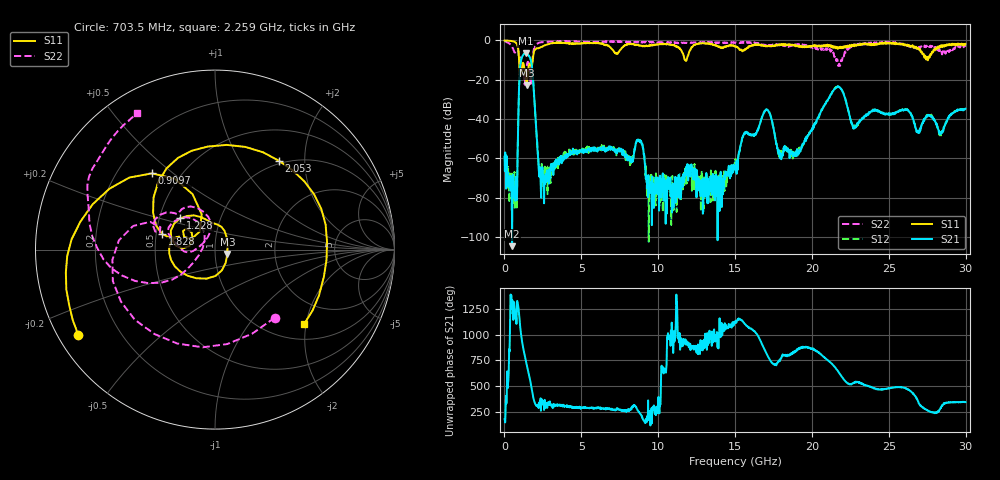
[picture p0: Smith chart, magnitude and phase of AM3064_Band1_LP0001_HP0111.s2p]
# Hz S DB R 50.0
!freq dBS11 angS11 dBS21 angS21 dBS12 angS12 dBS22 angS22
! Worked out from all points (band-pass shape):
!   1600 points, 10 MHz to 29.98 GHz, reference 50 ohm
!   highest |S21| = -6.51 dB at 1.378 GHz (marker M1); lowest = -104.6 dB at 497.3 MHz (marker M2)
!   |S21| within 3 dB of the highest: 1.094 GHz to 1.698 GHz (603.7 MHz wide, 43.2 % of centre)
!   lowest |S11| = -22.7 dB at 1.453 GHz (marker M3), VSWR 1.16, Z = 57.3 - j2.79 ohm
!   |S11| at or under -10 dB: 949.3 MHz to 1.833 GHz (883.2 MHz wide, 63.5 % of centre); 11.74 GHz to 11.84 GHz (102.1 MHz wide, 0.866 % of centre); 27.53434 GHz to 27.54646 GHz (12.12 MHz wide, 0.044 % of centre)
!   |S22| runs from -23.1 to -0.2 dB; largest |S21 - S12| = 0.0045
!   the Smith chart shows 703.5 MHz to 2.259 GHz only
!   S11 on the Smith chart (normalised r, x): 703.5 MHz: 0.06, -0.29; 909.7 MHz: 0.35, +0.42; 1.228 GHz: 0.64, +0.24; 1.828 GHz: 0.54, +0.10; 2.053 GHz: 0.95, +1.50; 2.259 GHz: 1.36, -1.95
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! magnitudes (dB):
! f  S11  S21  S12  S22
! 10 MHz  -0.1  -59.1  -58.7  -0.2
! 497.3 MHz  -0.4  -104.6  -67.3  -3.2
! 703.5 MHz  -0.9  -81.6  -73.1  -5.9
! 909.7 MHz  -5.2  -36.3  -36.2  -6.5
! 1.228 GHz  -11.7  -7.3  -7.3  -13.1
! 1.378 GHz  -17.6  -6.5  -6.5  -16.4
! 1.453 GHz  -22.7  -6.7  -6.7  -12.8
! 1.828 GHz  -10.3  -16.4  -16.3  -9.1
! 2.053 GHz  -4.3  -43.4  -43.3  -2.0
! 2.259 GHz  -3.8  -69.2  -67.0  -1.1
! 5.015 GHz  -1.4  -56.5  -56.1  -0.6
! 8.763 GHz  -2.7  -50.9  -51.0  -1.1
! 10 GHz  -2.0  -78.3  -71.9  -0.9
! 15 GHz  -3.0  -65.8  -63.8  -1.2
! 17.01 GHz  -3.1  -35.2  -35.2  -2.4
! 17.97 GHz  -2.4  -57.8  -58.3  -2.0
! 19.99 GHz  -3.2  -45.9  -45.7  -3.3
! 21.66 GHz  -3.7  -23.6  -23.4  -10.0
! 22.75 GHz  -2.9  -44.7  -43.6  -1.9
! 25 GHz  -1.1  -37.7  -37.4  -1.1
! 28.39 GHz  -2.7  -46.9  -48.3  -5.1
! 29.98 GHz  -1.8  -34.8  -35.0  -3.2
